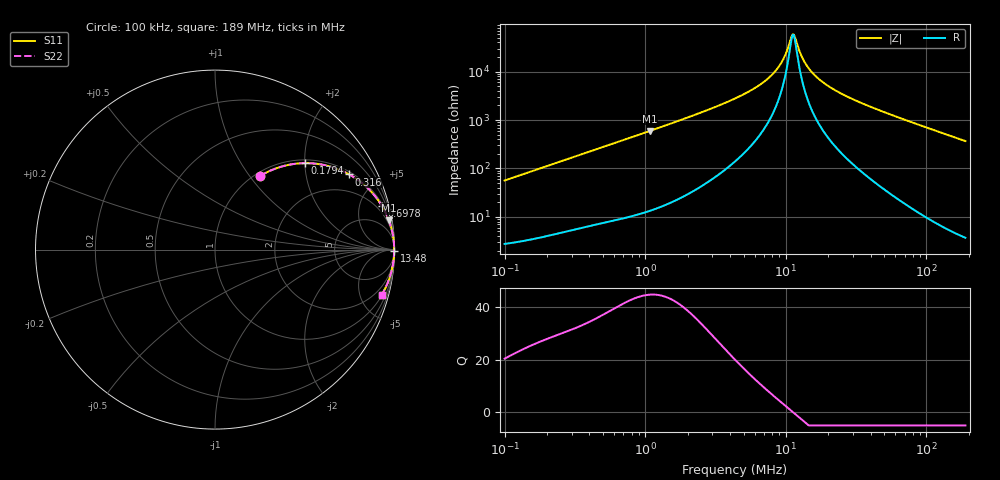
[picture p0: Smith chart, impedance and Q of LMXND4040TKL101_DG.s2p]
! LMXND4040TKL101_DG  S-PARAMETER MODEL  ( General Type )
! Model Generated by TAIYO YUDEN Corporation (https://www.yuden.co.jp/en/)
! Version 1.0
! TAIYO YUDEN Control No. 191023NI43SB-FBB
! Copyright(c) 2019 TAIYO YUDEN CO.,LTD. All Rights Reserved.
! Product Description (link to TY-COMPAS)
! https://ds.yuden.co.jp/TYCOMPAS/or/detail?pn=LMXND4040TKL101MDG&u=M
! Products Name : Inductors
! Characteristics :
!  Inductance : 100 uH , SRF(min) : 6.5 MHz , DC Resistance(max) : 1.74 Ohm
!  Rated Current : Saturation :420 mA , Temp Rise : 280 mA (40 degC)
!  Case Size : 4.0 x 4.0 / 0.157 x 0.157 [mm/inch] , Thickness : 1.8 / 0.071 [mm/inch]
!  (Conditions: Temperature = 25 degC , DC Bias Current/Voltage = 0A / 0V)
! External Node Assignments :
!  1  o---GGG---o  2
! GND o---------o GND
! Frequency Range : 0.1MHz  -  189.042664MHz  [ 402 STEP ]
# MHz S RI R 50
! Freq[MHz].  S11 Real  S11 Imag  S21 Real  S21 Imag  S12 Real  S12 Imag  S22 Real  S22 Imag
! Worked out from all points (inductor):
!   401 points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, 100 kHz to 189 MHz, reference 50 ohm
!   read as one part in series: L = 89.3 uH near 103.8 kHz
!   highest Q = 44.7 at 1.077 MHz (marker M1), where L = 87.8 uH
!   self-resonance near 11.16 MHz
!   S11 on the Smith chart (normalised r, x): 100 kHz: 1.06, +1.13; 179.4 kHz: 1.07, +2.01; 316 kHz: 1.11, +3.50; 697.8 kHz: 1.19, +7.68; 13.48 MHz: open; 189 MHz: 1.07, -7.35
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0.1  0.2514 0.41  0.7486 -0.41  0.7486 -0.41  0.2514 0.41
0.179446  0.5019 0.4817  0.4981 -0.4817  0.4981 -0.4817  0.5019 0.4817
0.315991  0.7478 0.4189  0.2522 -0.4189  0.2522 -0.4189  0.7478 0.4189
0.353854  0.7864 0.395  0.2136 -0.395  0.2136 -0.395  0.7864 0.395
0.697773  0.9314 0.2409  0.0686 -0.2409  0.0686 -0.2409  0.9314 0.2409
1.076754  0.969 0.1625  0.031 -0.1625  0.031 -0.1625  0.969 0.1625
1.252125  0.9766 0.1405  0.0234 -0.1405  0.0234 -0.1405  0.9766 0.1405
4.347904  0.9969 0.0357  0.00307 -0.0357  0.00307 -0.0357  0.9969 0.0357
6.340272  0.9979 0.0197  0.00211 -0.0197  0.00211 -0.0197  0.9979 0.0197
8.102072  0.9982 0.0109  0.00182 -0.0109  0.00182 -0.0109  0.9982 0.0109
9.421657  0.9983 0.00583  0.00172 -0.00583  0.00172 -0.00583  0.9983 0.00583
9.970145  0.9983 0.00397  0.0017 -0.00397  0.0017 -0.00397  0.9983 0.00397
10.75145  0.9983 0.00151  0.00168 -0.00151  0.00168 -0.00151  0.9983 0.00151
11.16477  0.9983 0.00029  0.00168 -0.00029  0.00168 -0.00029  0.9983 0.00029
11.59398  0.9983 -0.000934  0.00168 0.000934  0.00168 0.000934  0.9983 -0.000934
12.74059  0.9983 -0.004  0.00169 0.004  0.00169 0.004  0.9983 -0.004
13.4823  0.9983 -0.00586  0.00171 0.00586  0.00171 0.00586  0.9983 -0.00586
15.38522  0.9982 -0.0103  0.00178 0.0103  0.00178 0.0103  0.9982 -0.0103
18.5788  0.998 -0.0169  0.00196 0.0169  0.00196 0.0169  0.998 -0.0169
23.74138  0.9976 -0.0265  0.00238 0.0265  0.00238 0.0265  0.9976 -0.0265
54.44117  0.9926 -0.0746  0.00736 0.0746  0.00736 0.0746  0.9926 -0.0746
189.0427  0.9288 -0.2521  0.0712 0.2521  0.0712 0.2521  0.9288 -0.2521
